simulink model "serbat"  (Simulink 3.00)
settings: Solver=ode45  StartTime=0.0  StopTime=2  MaxStep=0.01  RelTol=1e-5  AbsTol=1e-5
undefined symbols (not defined in the file or in its folder): A, dbar, hiniz, k, mu, tau, td

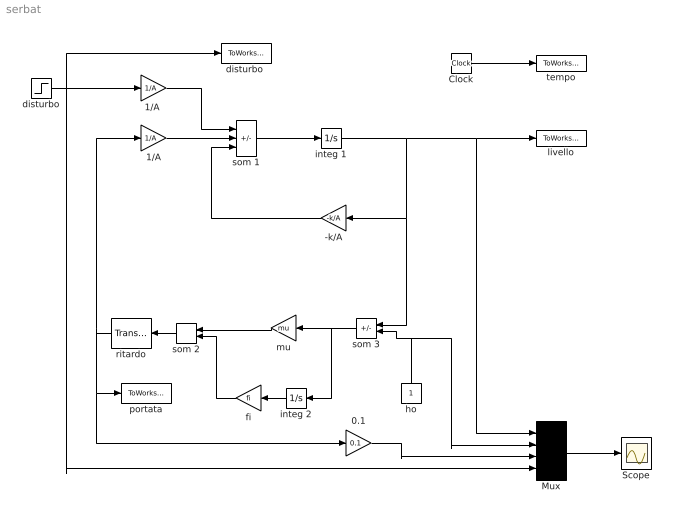
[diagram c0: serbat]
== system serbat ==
  -k/A : Gain  Orientation=left  Gain=-k/A  SaturateOnIntegerOverflow=on
  0.1 : Gain  Gain=0.1  SaturateOnIntegerOverflow=on
  1/A : Gain  Gain=1/A  SaturateOnIntegerOverflow=on
  "1/A " : Gain  Gain=1/A  SaturateOnIntegerOverflow=on
  Clock : Clock
  Mux : Mux  Inputs=4
  Scope : Scope
  disturbo : Step  Time=td  Before=0  After=dbar  SampleTime=0
  "disturbo " : ToWorkspace  VariableName=d  SampleTime=0  SaveFormat=Matrix
  fi : Gain  Orientation=left  Gain=fi  SaturateOnIntegerOverflow=on
  ho : Constant  Orientation=up  Value=1
  integ 1 : Integrator  ExternalReset=none  InitialConditionSource=internal  InitialCondition=hiniz  LimitOutput=off  UpperSaturationLimit=inf  LowerSaturationLimit=-inf  ShowSaturationPort=off  ShowStatePort=off  AbsoluteTolerance=auto
  integ 2 : Integrator  Orientation=left  ExternalReset=none  InitialConditionSource=internal  InitialCondition=0  LimitOutput=off  UpperSaturationLimit=inf  LowerSaturationLimit=-inf  ShowSaturationPort=off  ShowStatePort=off  AbsoluteTolerance=auto
  livello : ToWorkspace  VariableName=h  SampleTime=0  SaveFormat=Matrix
  mu : Gain  Orientation=left  Gain=mu  SaturateOnIntegerOverflow=on
  portata : ToWorkspace  VariableName=qe  SampleTime=0  SaveFormat=Matrix
  ritardo : TransportDelay  Orientation=left  DelayTime=tau  InitialInput=0  BufferSize=1024
  som 1 : Sum  Inputs=-++  SaturateOnIntegerOverflow=on
  som 2 : Sum  Orientation=left  Inputs=++  SaturateOnIntegerOverflow=on
  som 3 : Sum  Orientation=left  Inputs=-+  SaturateOnIntegerOverflow=on
  tempo : ToWorkspace  VariableName=t  SampleTime=0  SaveFormat=Matrix
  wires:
  som 1/1 -> integ 1/1
  Clock/1 -> tempo/1
  -k/A/1 -> som 1/3
  1/A/1 -> som 1/2
  "1/A "/1 -> som 1/1
  som 3/1 -> mu/1, integ 2/1
  mu/1 -> som 2/1
  som 2/1 -> ritardo/1
  integ 2/1 -> fi/1
  fi/1 -> som 2/2
  ho/1 -> som 3/2, Mux/2
  ritardo/1 -> 1/A/1, 0.1/1, portata/1
  Mux/1 -> Scope/1
  disturbo/1 -> "1/A "/1, Mux/4, "disturbo "/1
  0.1/1 -> Mux/3
  integ 1/1 -> -k/A/1, som 3/1, Mux/1, livello/1
